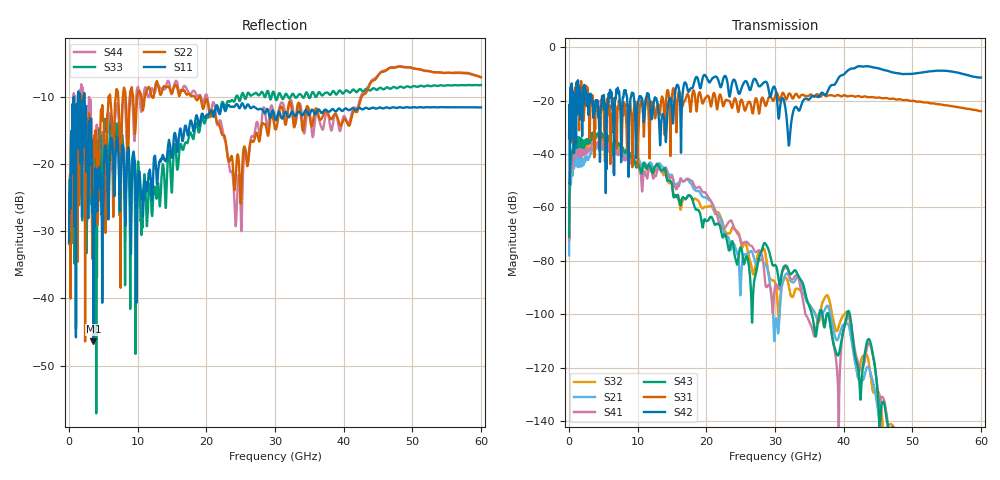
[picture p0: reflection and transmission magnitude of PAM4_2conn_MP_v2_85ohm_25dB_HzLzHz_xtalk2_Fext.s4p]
! Info: Touchstone file created by Circ.  Input file=FAB50GbE_2conn_Midplane_Examax_Topo2_v2_85ohm_25dB_HzLzHz.circ
# Hz S RI R 50
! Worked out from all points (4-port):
!   6000 points, 10 MHz to 60 GHz, reference 50 ohm
!   strongest paths, dB at 10 MHz, 15.01 GHz, 30.01 GHz, 45.01 GHz, 60 GHz:
!     S42: -34.0, -24.0, -15.3, -7.9, -11.4
!     S31: -33.9, -17.8, -18.3, -18.9, -24.0
!     S43: -71.0, -51.7, -81.6, -130.9, -180.3
!     S41: -72.5, -48.6, -89.8, -130.1, -187.4
!     S21: -78.0, -48.0, -104.1, -135.9, -184.8
!     S32: -72.5, -51.5, -88.2, -128.9, -170.7
!   lowest |S11| = -46.4 dB at 3.56 GHz (marker M1), VSWR 1.01, Z = 50.5 + j0.128 ohm
!   |S11| at or under -10 dB: start of sweep to 673.1 MHz; 682.6 MHz to 1.3 GHz (617.3 MHz wide, 62.3 % of centre); 2.243 GHz to end of sweep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
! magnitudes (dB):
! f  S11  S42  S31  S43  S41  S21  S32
! 10 MHz  -31.6  -34.0  -33.9  -71.0  -72.5  -78.0  -72.5
! 820 MHz  -14.8  -26.7  -17.6  -34.3  -37.2  -40.6  -36.2
! 3.56 GHz  -46.4  -26.0  -24.1  -32.3  -35.6  -37.9  -33.6
! 24.41 GHz  -11.0  -14.5  -21.0  -80.8  -69.3  -76.4  -68.6
! 32.06 GHz  -13.0  -36.5  -17.4  -84.3  -85.1  -86.0  -90.0
! 42.09 GHz  -11.7  -7.2  -18.3  -119.8  -117.9  -123.5  -123.6
! 60 GHz  -11.6  -11.4  -24.0  -180.3  -187.4  -184.8  -170.7
